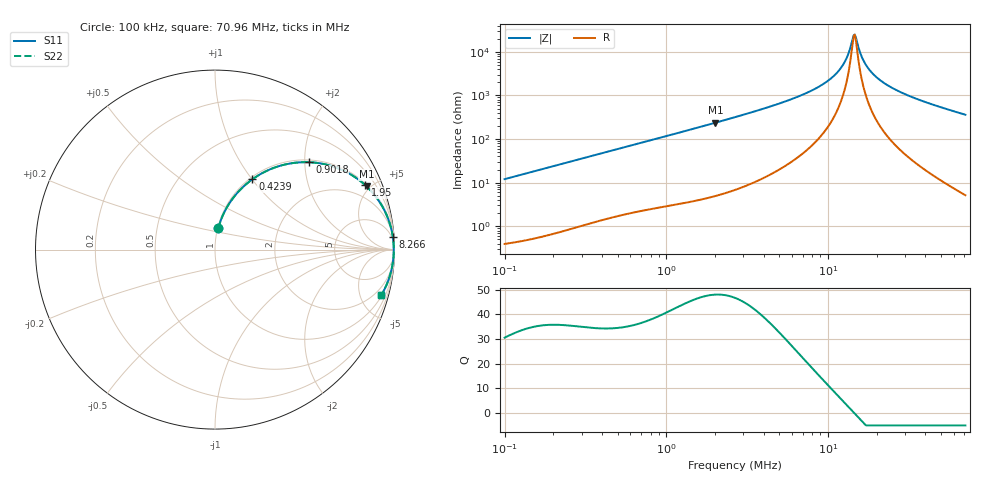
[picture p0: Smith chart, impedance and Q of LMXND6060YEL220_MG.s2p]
! LMXND6060YEL220_MG  S-PARAMETER MODEL  ( General Type )
! Model Generated by TAIYO YUDEN Corporation (https://www.yuden.co.jp/en/)
! Version 1.0
! TAIYO YUDEN Control No. 191025NI43SB-FBB
! Copyright(c) 2019 TAIYO YUDEN CO.,LTD. All Rights Reserved.
! Product Description (link to TY-COMPAS)
! https://ds.yuden.co.jp/TYCOMPAS/or/detail?pn=LMXND6060YEL220MMG&u=M
! Products Name : Inductors
! Characteristics :
!  Inductance : 22 uH , SRF(min) : 7.0 MHz , DC Resistance(max) : 0.1391 Ohm
!  Rated Current : Saturation :2000 mA , Temp Rise : 1600 mA (40 degC)
!  Case Size : 6.0 x 6.0 / 0.236 x 0.236 [mm/inch] , Thickness : 4.5 / 0.177 [mm/inch]
!  (Conditions: Temperature = 25 degC , DC Bias Current/Voltage = 0A / 0V)
! External Node Assignments :
!  1  o---GGG---o  2
! GND o---------o GND
! Frequency Range : 0.1MHz  -  70.9631MHz  [ 402 STEP ]
# MHz S RI R 50
! Freq[MHz].  S11 Real  S11 Imag  S21 Real  S21 Imag  S12 Real  S12 Imag  S22 Real  S22 Imag
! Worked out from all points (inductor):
!   401 points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, 100 kHz to 70.96 MHz, reference 50 ohm
!   read as one part in series: L = 19.1 uH near 103.3 kHz
!   highest Q = 48 at 2.015 MHz (marker M1), where L = 18.7 uH
!   self-resonance near 14.44 MHz
!   S11 on the Smith chart (normalised r, x): 100 kHz: 1.01, +0.24; 423.9 kHz: 1.03, +1.00; 901.8 kHz: 1.05, +2.11; 1.95 MHz: 1.10, +4.59; 8.266 MHz: 3, +28; 70.96 MHz: 1.10, -7.24
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0.1  0.018 0.1177  0.982 -0.1177  0.982 -0.1177  0.018 0.1177
0.300295  0.1203 0.3114  0.8797 -0.3114  0.8797 -0.3114  0.1203 0.3114
0.423865  0.2079 0.3915  0.7921 -0.3915  0.7921 -0.3915  0.2079 0.3915
0.90177  0.5258 0.4868  0.4742 -0.4868  0.4742 -0.4868  0.5258 0.4868
1.950259  0.8353 0.3606  0.1647 -0.3606  0.1647 -0.3606  0.8353 0.3606
2.015336  0.8442 0.3524  0.1558 -0.3524  0.1558 -0.3524  0.8442 0.3524
2.70797  0.9079 0.2786  0.0921 -0.2786  0.0921 -0.2786  0.9079 0.2786
5.135935  0.9743 0.1435  0.0257 -0.1435  0.0257 -0.1435  0.9743 0.1435
7.999526  0.9902 0.0748  0.00981 -0.0748  0.00981 -0.0748  0.9902 0.0748
8.266457  0.9909 0.0704  0.00913 -0.0704  0.00913 -0.0704  0.9909 0.0704
10.23241  0.9941 0.0427  0.00586 -0.0427  0.00586 -0.0427  0.9941 0.0427
11.86113  0.9954 0.0247  0.00459 -0.0247  0.00459 -0.0247  0.9954 0.0247
12.8755  0.9958 0.0149  0.00418 -0.0149  0.00418 -0.0149  0.9958 0.0149
14.20789  0.9961 0.00327  0.00394 -0.00327  0.00394 -0.00327  0.9961 0.00327
14.68198  0.9961 -0.0006  0.00393 0.0006  0.00393 0.0006  0.9961 -0.0006
15.1719  0.9961 -0.00447  0.00394 0.00447  0.00394 0.00447  0.9961 -0.00447
16.20131  0.9959 -0.0122  0.00406 0.0122  0.00406 0.0122  0.9959 -0.0122
17.58685  0.9956 -0.022  0.00438 0.022  0.00438 0.022  0.9956 -0.022
20.05436  0.9947 -0.0379  0.00533 0.0379  0.00533 0.0379  0.9947 -0.0379
24.02217  0.9924 -0.0608  0.0076 0.0608  0.0076 0.0608  0.9924 -0.0608
37.41596  0.98 -0.1258  0.02 0.1258  0.02 0.1258  0.98 -0.1258
70.9631  0.926 -0.2548  0.074 0.2548  0.074 0.2548  0.926 -0.2548
